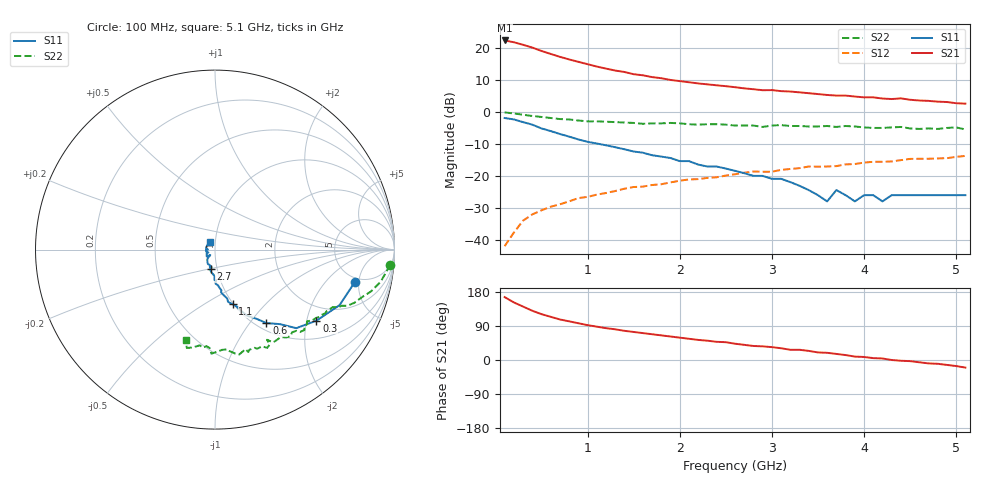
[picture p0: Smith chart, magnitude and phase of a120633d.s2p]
!  INA-12063 S PARAMETERS
!  Vd = 3 V  Id = 8 mA  LAST UPDATED 10-07-96
# ghz s ma r 50
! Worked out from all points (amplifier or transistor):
!   51 points, 100 MHz to 5.1 GHz, reference 50 ohm
!   highest |S21| = 22.3 dB at 100 MHz (marker M1)
!   |S21| within 3 dB of that: start of sweep to 473.9 MHz
!   unconditionally stable (mu >= 1): 923.7 MHz to end of sweep
!   at 900 MHz: K = 0.98, MSG = 21.3 dB, |S12| = -26.9 dB
!   at 2.6 GHz: K = 1.37, MAG = 10.0 dB, |S12| = -19.5 dB
!   at 5.1 GHz: K = 1.42, MAG = 4.3 dB, |S12| = -13.8 dB
!   S11 on the Smith chart (normalised r, x): 100 MHz: 4.44, -4.44; 300 MHz: 1.52, -2.29; 600 MHz: 1.11, -1.21; 1.1 GHz: 0.99, -0.67; 2.7 GHz: 0.93, -0.20; 5.1 GHz: 0.95, +0.08
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0.1  0.8 -13.0  12.97 166.0  0.008 73.0  0.98 -5.0
0.2  0.76 -24.0  12.17 152.0  0.013 72.0  0.94 -11.0
0.3  0.69 -35.0  11.1 141.0  0.02 75.0  0.9 -15.0
0.4  0.63 -44.0  10.06 130.0  0.025 69.0  0.86 -18.0
0.5  0.55 -49.0  8.89 121.0  0.029 64.0  0.83 -21.0
0.6  0.5 -55.0  8 114.0  0.033 64.0  0.8 -23.0
0.7  0.45 -59.0  7.2 107.0  0.036 59.0  0.77 -24.0
0.8  0.41 -64.0  6.56 102.0  0.04 59.0  0.76 -25.0
1  0.34 -69.0  5.53 92.0  0.047 58.0  0.71 -29.0
1.1  0.32 -72.0  5.08 88.0  0.051 57.0  0.71 -30.0
1.4  0.26 -79.0  4.18 77.0  0.063 53.0  0.68 -34.0
1.5  0.24 -82.0  3.86 74.0  0.067 53.0  0.67 -36.0
1.8  0.2 -85.0  3.34 65.0  0.074 51.0  0.66 -41.0
2.2  0.15 -91.0  2.77 53.0  0.089 44.0  0.63 -47.0
2.6  0.12 -102.0  2.42 43.0  0.106 42.0  0.61 -53.0
2.7  0.11 -103.0  2.32 40.0  0.112 41.0  0.61 -56.0
3.5  0.05 -130.0  1.89 20.0  0.139 27.0  0.59 -71.0
3.6  0.04 -131.0  1.83 19.0  0.14 25.0  0.6 -72.0
3.7  0.06 -140.0  1.79 16.0  0.142 26.0  0.58 -73.0
3.9  0.04 -156.0  1.73 9.0  0.153 25.0  0.59 -79.0
4.3  0.05 171.0  1.58 0.0  0.168 17.0  0.57 -89.0
5.1  0.05 122.0  1.34 -20.0  0.205 6.0  0.53 -108.0
